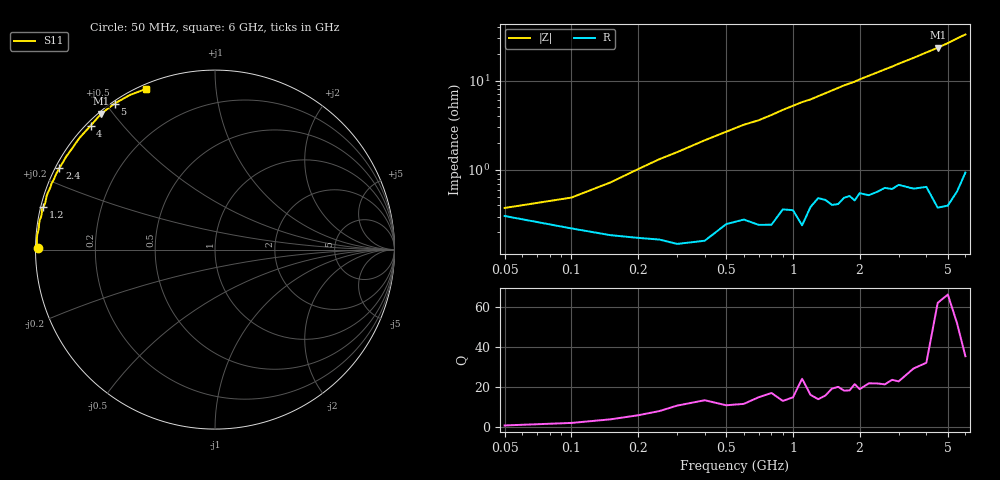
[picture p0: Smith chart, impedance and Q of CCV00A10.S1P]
! Infineon Technologies  Discrete & RF Semiconductors
! BBY57-02W
! Si Tuning Diode in SCD-80
! VR = 0
! S-Parameters:  June  2000
# GHz  S  MA  R  50
!  f  S11
! GHz  MAG  ANG
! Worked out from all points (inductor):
!   34 points, 50 MHz to 6 GHz, reference 50 ohm
!   read as one part to ground: L = 799 pH near 150 MHz
!   highest Q = 61.9 at 4.5 GHz (marker M1), where L = 825 pH
!   S11 on the Smith chart (normalised r, x): 50 MHz: 0.01, +0.00; 1.2 GHz: 0.01, +0.12; 2.4 GHz: 0.01, +0.25; 4 GHz: 0.01, +0.41; 5 GHz: 0.01, +0.53; 6 GHz: 0.02, +0.66
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0.05  0.9879 179.5
0.15  0.9926 178.4
0.3  0.9941 176.4
0.4  0.9936 175.1
0.6  0.989 172.7
0.7  0.9904 171.8
0.8  0.9904 170.6
0.9  0.9858 169.3
1  0.9861 168.1
1.1  0.9906 166.9
1.2  0.985 166.0
1.3  0.9812 164.8
1.5  0.9843 162.4
1.6  0.984 161.2
1.7  0.9813 160.0
1.8  0.9805 159.0
1.9  0.9826 158.0
2  0.9792 156.7
2.2  0.9804 154.5
2.4  0.9788 152.3
2.8  0.9777 148.0
3  0.9755 145.7
3.5  0.9784 140.5
4  0.9782 135.1
4.5  0.9877 130.0
5  0.9876 124.5
5.5  0.9832 118.7
6  0.9743 113.4
